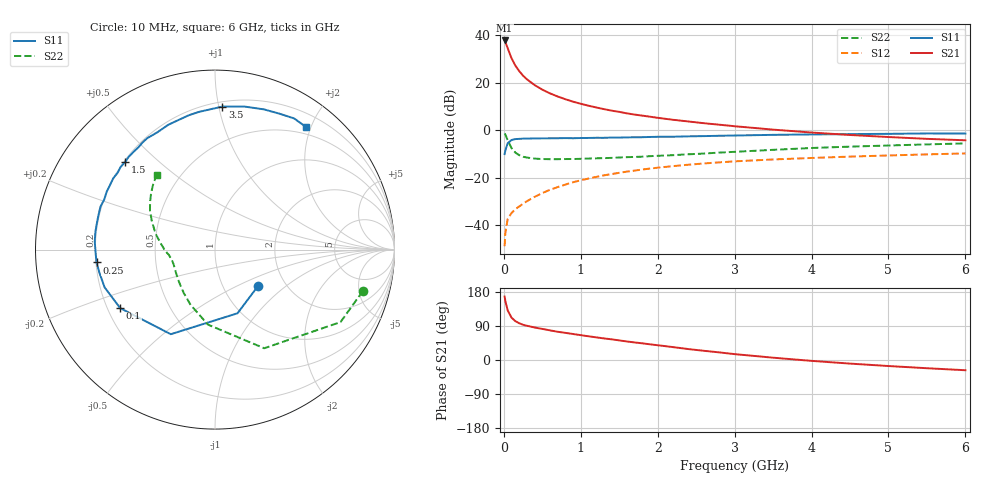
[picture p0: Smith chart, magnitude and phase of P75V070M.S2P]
! SIEMENS Small Signal Semiconductors
! BFP196
! Si NPN RF Bipolar Junction Transistor in SOT143
! VCE = 5 V  IC = 70 mA
! Common Emitter S-Parameters:  May  1996
# GHz  S  MA  R  50
!  f  S11  S21  S12  S22
! GHz  MAG  ANG  MAG  ANG  MAG  ANG  MAG  ANG
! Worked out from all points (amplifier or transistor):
!   36 points, 10 MHz to 6 GHz, reference 50 ohm
!   highest |S21| = 37.8 dB at 10 MHz (marker M1)
!   |S21| within 3 dB of that: start of sweep to 46.87 MHz
!   unconditionally stable (mu >= 1): 415.4 MHz to 4.814 GHz
!   at 250 MHz: K = 0.87, MSG = 27.0 dB, |S12| = -31.0 dB
!   at 1.4 GHz: K = 1.08, MAG = 11.6 dB, |S12| = -18.5 dB
!   at 6 GHz: K = 0.99, MSG = 2.8 dB, |S12| = -9.8 dB
!   S11 on the Smith chart (normalised r, x): 10 MHz: 1.46, -0.66; 100 MHz: 0.25, -0.27; 250 MHz: 0.20, -0.05; 1.5 GHz: 0.21, +0.39; 3.5 GHz: 0.23, +1.03; 6 GHz: 0.39, +1.93
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0.01  0.3141 -40.2  77.8 167.4  0.0036 80.1  0.8553 -15.7
0.02  0.3763 -70.5  72 155.2  0.0069 71.4  0.8076 -30.0
0.05  0.5319 -117.6  53.39 130.9  0.0135 55.5  0.6142 -63.5
0.1  0.6208 -148.3  32.79 111.7  0.018 49.7  0.4196 -95.4
0.15  0.65 -161.1  22.93 102.5  0.0217 51.3  0.3367 -113.8
0.2  0.6565 -168.4  17.57 97.0  0.0247 54.4  0.2978 -125.8
0.25  0.6638 -173.8  14.08 93.0  0.0283 56.3  0.2756 -134.9
0.3  0.665 -177.9  11.82 90.3  0.0319 59.2  0.2648 -140.8
0.4  0.6716 176.1  8.94 85.8  0.0394 61.7  0.2522 -149.9
0.5  0.6737 171.6  7.157 82.0  0.0473 63.2  0.2466 -155.6
0.6  0.6745 167.1  5.966 78.2  0.0556 64.0  0.2451 -159.5
0.7  0.6774 163.1  5.133 74.5  0.0633 64.0  0.2452 -162.5
0.9  0.6775 155.6  3.991 68.6  0.0801 62.5  0.247 -167.1
1.1  0.6865 148.5  3.283 62.6  0.0957 60.8  0.2526 -170.2
1.5  0.6991 135.8  2.435 51.7  0.1266 55.6  0.2657 -175.4
1.7  0.7094 129.4  2.134 46.3  0.1408 52.7  0.2733 -178.4
2.2  0.7283 116.1  1.657 34.0  0.1751 45.2  0.2978 175.2
2.8  0.7629 100.9  1.306 20.1  0.21 36.3  0.3376 166.0
3.5  0.7982 87.0  1.028 6.1  0.2418 26.2  0.3859 155.8
4.5  0.8274 70.8  0.793 -9.5  0.2777 14.2  0.4504 143.4
5.5  0.8534 58.9  0.657 -21.7  0.3092 3.6  0.5023 133.2
6  0.8508 53.4  0.613 -27.0  0.324 -2.1  0.5269 128.2
